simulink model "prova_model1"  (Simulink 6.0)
settings: Solver=ode45  StartTime=0.0  StopTime=30.0  RelTol=1e-3
libraries: simulink x1

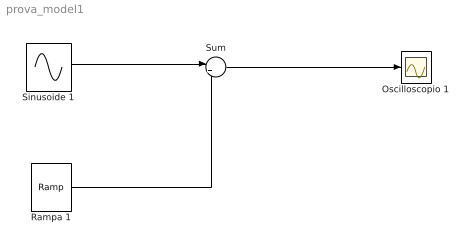
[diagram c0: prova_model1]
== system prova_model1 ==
  Oscilloscopio 1 : Scope
  Rampa 1 : simulink/Sources/Ramp  slope=0.25  start=0  X0=0
  Sinusoide 1 : Sin  Amplitude=3  Frequency=0.2*pi  Phase=pi  SampleTime=0.01
  Sum : Sum  Inputs=|++
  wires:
  Sinusoide 1/1 -> Sum/1
  Rampa 1/1 -> Sum/2
  Sum/1 -> Oscilloscopio 1/1
